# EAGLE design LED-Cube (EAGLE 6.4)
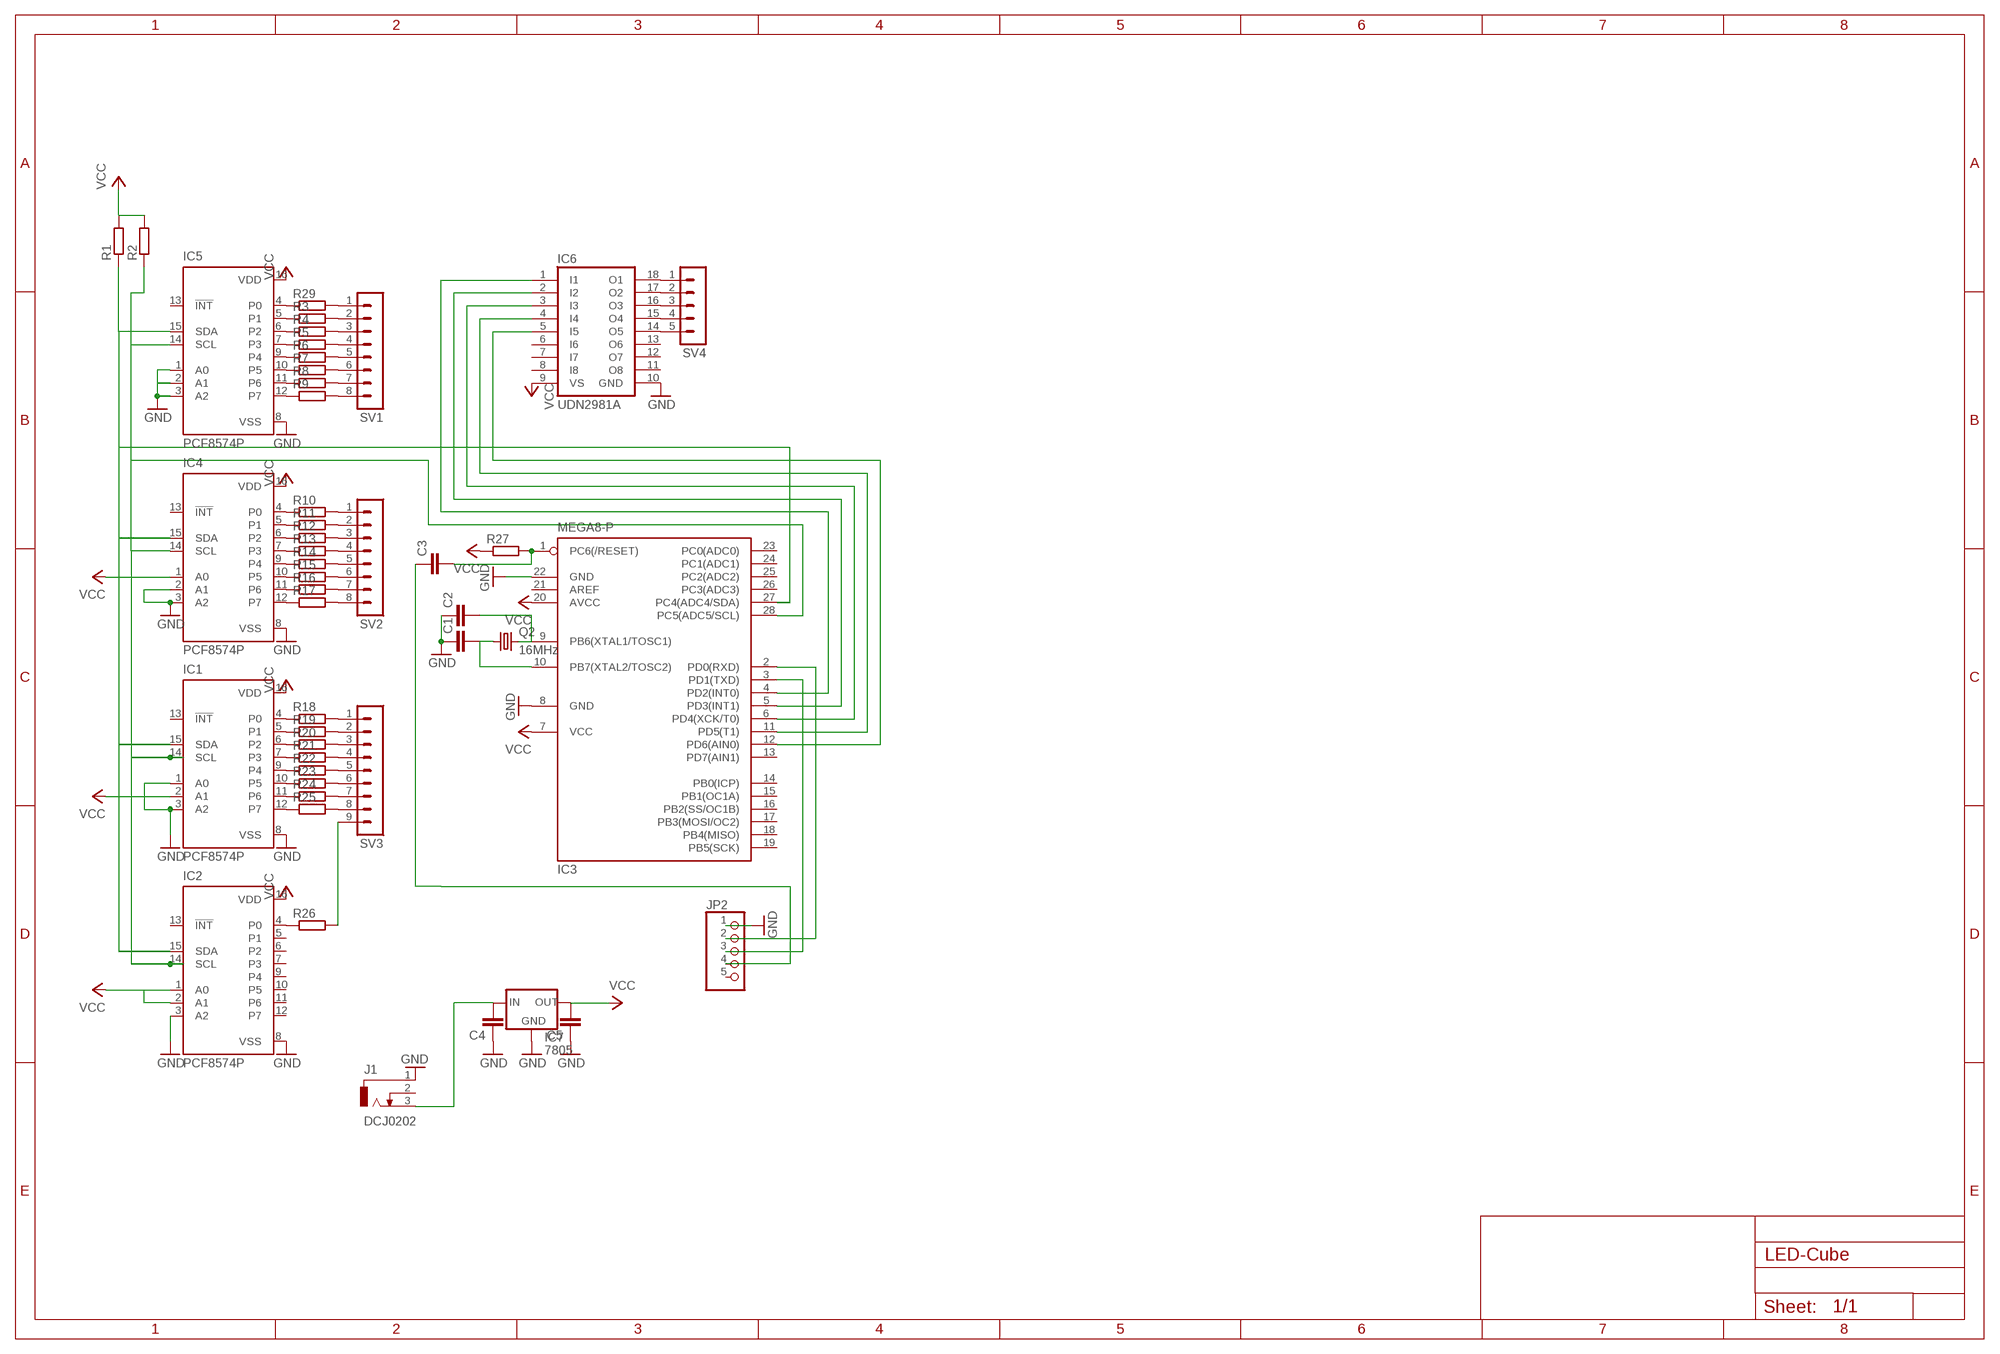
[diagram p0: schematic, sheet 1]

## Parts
C1  C-EU025-030X050  [C025-030X050]
C2  C-EU025-030X050  [C025-030X050]
C3  C-EU025-030X050  [C025-030X050]
C4  C-EU025-030X050  [C025-030X050]
C5  C-EU025-030X050  [C025-030X050]
IC1  PCF8574P  [DIL16]
IC2  PCF8574P  [DIL16]
IC3  MEGA8-P  [DIL28-3]
IC4  PCF8574P  [DIL16]
IC5  PCF8574P  [DIL16]
IC6  UDN2981A  [DIL18]
IC7  7805  V_REG_78XXSIDE  [78XXL]
J1  DCJ0202  [DCJ0202]
JP2  PINHD-1X5  [1X05]
Q2  16MHz  CRYSTALHC49S  [HC49/S]
R1  R-EU_0204/7  [0204/7]
R2  R-EU_0204/7  [0204/7]
R3  R-EU_0207/7  [0207/7]
R4  R-EU_0207/7  [0207/7]
R5  R-EU_0207/7  [0207/7]
R6  R-EU_0207/7  [0207/7]
R7  R-EU_0207/7  [0207/7]
R8  R-EU_0207/7  [0207/7]
R9  R-EU_0207/7  [0207/7]
R10  R-EU_0207/7  [0207/7]
R11  R-EU_0207/7  [0207/7]
R12  R-EU_0207/7  [0207/7]
R13  R-EU_0207/7  [0207/7]
R14  R-EU_0207/7  [0207/7]
R15  R-EU_0207/7  [0207/7]
R16  R-EU_0207/7  [0207/7]
R17  R-EU_0207/7  [0207/7]
R18  R-EU_0207/7  [0207/7]
R19  R-EU_0207/7  [0207/7]
R20  R-EU_0207/7  [0207/7]
R21  R-EU_0207/7  [0207/7]
R22  R-EU_0207/7  [0207/7]
R23  R-EU_0207/7  [0207/7]
R24  R-EU_0207/7  [0207/7]
R25  R-EU_0207/7  [0207/7]
R26  R-EU_0207/7  [0207/7]
R27  R-EU_0207/7  [0207/7]
R29  R-EU_0207/7  [0207/7]
SV1  MA08-1  [MA08-1]
SV2  MA08-1  [MA08-1]
SV3  MA09-1  [MA09-1]
SV4  MA05-1  [MA05-1]

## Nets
GND [GND]: C1.1 C2.1 C4.1 C5.1 IC1.1(A0) IC1.3(A2) IC1.8(VSS) IC2.3(A2) IC2.8(VSS) IC3.8(GND) IC3.22(GND) IC4.2(A1) IC4.3(A2) IC4.8(VSS) IC5.1(A0) IC5.2(A1) IC5.3(A2) IC5.8(VSS) IC6.10(GND) IC7.GND J1.1 JP2.1
N$1: IC1.14(SCL) IC2.14(SCL) IC3.28(PC5(ADC5/SCL)) IC4.14(SCL) IC5.14(SCL) R2.1
N$2: C3.1 JP2.4
N$3: IC5.4(P0) R29.1
N$4: R29.2 SV1.1
N$5: IC5.5(P1) R3.1
N$6: R3.2 SV1.2
N$7: IC5.6(P2) R4.1
N$8: R4.2 SV1.3
N$9: IC5.7(P3) R5.1
N$10: R5.2 SV1.4
N$11: IC5.10(P5) R7.1
N$12: R7.2 SV1.6
N$13: IC5.9(P4) R6.1
N$14: R6.2 SV1.5
N$15: IC5.11(P6) R8.1
N$16: R8.2 SV1.7
N$17: IC5.12(P7) R9.1
N$18: R9.2 SV1.8
N$19: IC4.4(P0) R10.1
N$20: R10.2 SV2.1
N$21: IC4.5(P1) R11.1
N$22: R11.2 SV2.2
N$23: IC4.6(P2) R12.1
N$24: R12.2 SV2.3
N$25: IC4.7(P3) R13.1
N$26: R13.2 SV2.4
N$27: IC4.9(P4) R14.1
N$28: R14.2 SV2.5
N$29: IC4.10(P5) R15.1
N$30: R15.2 SV2.6
N$31: IC4.11(P6) R16.1
N$32: R16.2 SV2.7
N$33: IC4.12(P7) R17.1
N$34: R17.2 SV2.8
N$35: IC1.4(P0) R18.1
N$36: R18.2 SV3.1
N$37: IC1.5(P1) R19.1
N$38: R19.2 SV3.2
N$39: IC1.6(P2) R20.1
N$40: R20.2 SV3.3
N$41: IC1.7(P3) R21.1
N$42: R21.2 SV3.4
N$43: IC1.9(P4) R22.1
N$44: R22.2 SV3.5
N$45: IC1.10(P5) R23.1
N$46: R23.2 SV3.6
N$47: IC1.11(P6) R24.1
N$48: R24.2 SV3.7
N$49: IC1.12(P7) R25.1
N$50: R25.2 SV3.8
N$51: IC2.4(P0) R26.1
N$52: R26.2 SV3.9
N$53: IC6.18(O1) SV4.1
N$54: IC6.17(O2) SV4.2
N$55: IC6.16(O3) SV4.3
N$56: IC6.15(O4) SV4.4
N$57: IC6.14(O5) SV4.5
N$59: IC3.3(PD1(TXD)) JP2.3
N$67: IC3.4(PD2(INT0)) IC6.1(I1)
N$68: IC3.5(PD3(INT1)) IC6.2(I2)
N$70: IC3.6(PD4(XCK/T0)) IC6.3(I3)
N$71: IC3.11(PD5(T1)) IC6.4(I4)
N$72: IC3.12(PD6(AIN0)) IC6.5(I5)
N$81: C3.2 IC3.1(PC6(/RESET)) R27.2
N$82: C2.2 IC3.9(PB6(XTAL1/TOSC1)) Q2.2
N$83: C1.2 IC3.10(PB7(XTAL2/TOSC2)) Q2.1
N$84: IC3.2(PD0(RXD)) JP2.2
N$86: C4.2 IC7.IN J1.3
N$88: IC1.15(SDA) IC2.15(SDA) IC3.27(PC4(ADC4/SDA)) IC4.15(SDA) IC5.15(SDA) R1.1
VCC [VCC]: C5.2 IC1.2(A1) IC1.16(VDD) IC2.1(A0) IC2.2(A1) IC2.16(VDD) IC3.7(VCC) IC3.20(AVCC) IC4.1(A0) IC4.16(VDD) IC5.16(VDD) IC6.9(VS) IC7.OUT R1.2 R2.2 R27.1
Unconnected: IC1.13(!INT) IC2.5(P1) IC2.6(P2) IC2.7(P3) IC2.9(P4) IC2.10(P5) IC2.11(P6) IC2.12(P7) IC2.13(!INT) IC3.13(PD7(AIN1)) IC3.14(PB0(ICP)) IC3.15(PB1(OC1A)) IC3.16(PB2(SS/OC1B)) IC3.17(PB3(MOSI/OC2)) IC3.18(PB4(MISO)) IC3.19(PB5(SCK)) IC3.21(AREF) IC3.23(PC0(ADC0)) IC3.24(PC1(ADC1)) IC3.25(PC2(ADC2)) IC3.26(PC3(ADC3)) IC4.13(!INT) IC5.13(!INT) IC6.6(I6) IC6.7(I7) IC6.8(I8) IC6.11(O8) IC6.12(O7) IC6.13(O6) J1.2 JP2.5

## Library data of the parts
C1-C5 = resistor:C-EU: CAPACITOR, European symbol
IC1 IC2 IC4 IC5 = micro-philips:PCF8574: I2C-Bus Remote 8-bit I/O expander http://www.semiconductors.philips.com/acrobat_download/datasheets/PCF8574_4.pdf; MPN: PCF8574PN; OC_FARNELL: 204020; OC_NEWARK: 11N8515
IC3 = atmel:MEGA8-P: MICROCONTROLLER 8 Kbytes FLASH, 1 kbytes SRAM, 512 bytes EEPROM, USART, 4-channel 10 bit ADC, 2-channel 8 bit ADC Pin compatible with Atmega48, ATMega88, ATMega168 Source: avr.lbr; OC_FARNELL: unknown; OC_NEWARK: unknown
IC6 = uln-udn:UDN298*: DRIVER ARRAY Source: Allegro Microsystems Inc. / UDN2981-UDN2984.pdf
IC7 = SparkFun:V_REG_78XX: Voltage Regulator Standard 7805 5V regulator. IGO (Input Ground Output). Spark Fun Electronics SKU : COM-00107
J1 = con-jack:DCJ0202: DC POWER JACK Source: DCJ0202.pdf; OC_FARNELL: unknown; OC_NEWARK: unknown
JP2 = pinhead:PINHD-1X5: PIN HEADER
Q2 = crystal:CRYSTAL: CRYSTAL; OC_FARNELL: 1667008; OC_NEWARK: unknown
R1 R2 = rcl:R-EU_: RESISTOR, European symbol
R3-R27 R29 = resistor:R-EU_: RESISTOR, European symbol
SV1 SV2 = con-lstb:MA08-1: PIN HEADER; OC_FARNELL: unknown; OC_NEWARK: unknown
SV3 = con-lstb:MA09-1: PIN HEADER; OC_FARNELL: unknown; OC_NEWARK: unknown
SV4 = con-lstb:MA05-1: PIN HEADER; OC_FARNELL: unknown; OC_NEWARK: unknown

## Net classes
1 VCC: width 0.508 mm
2 GND: width 0.508 mm

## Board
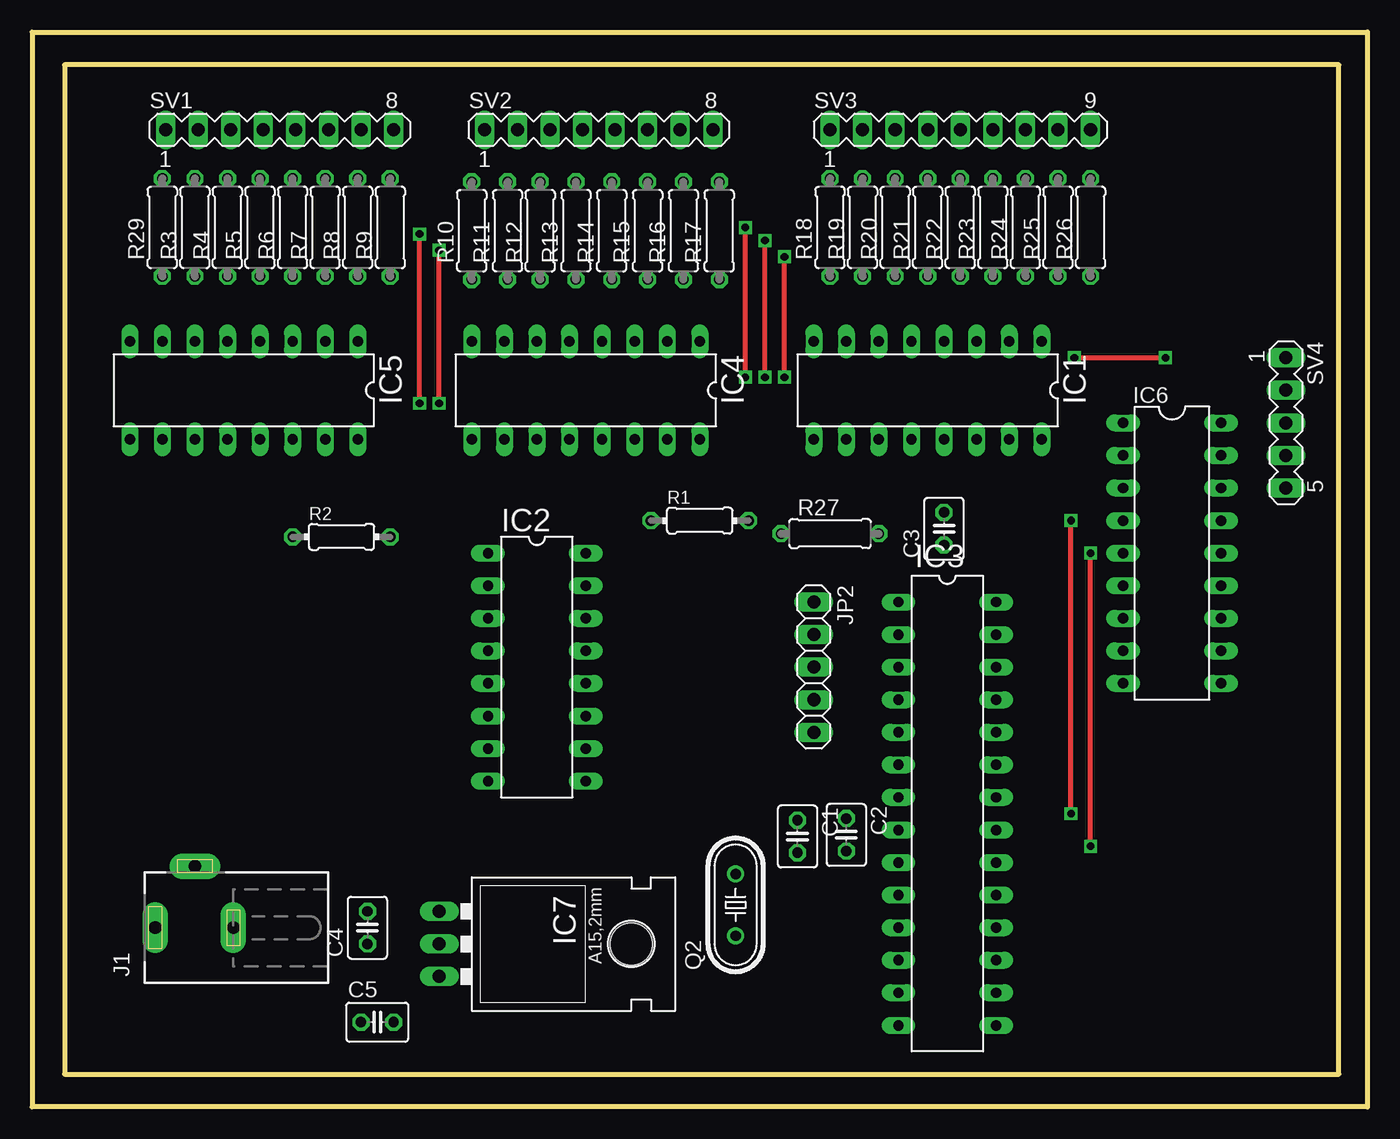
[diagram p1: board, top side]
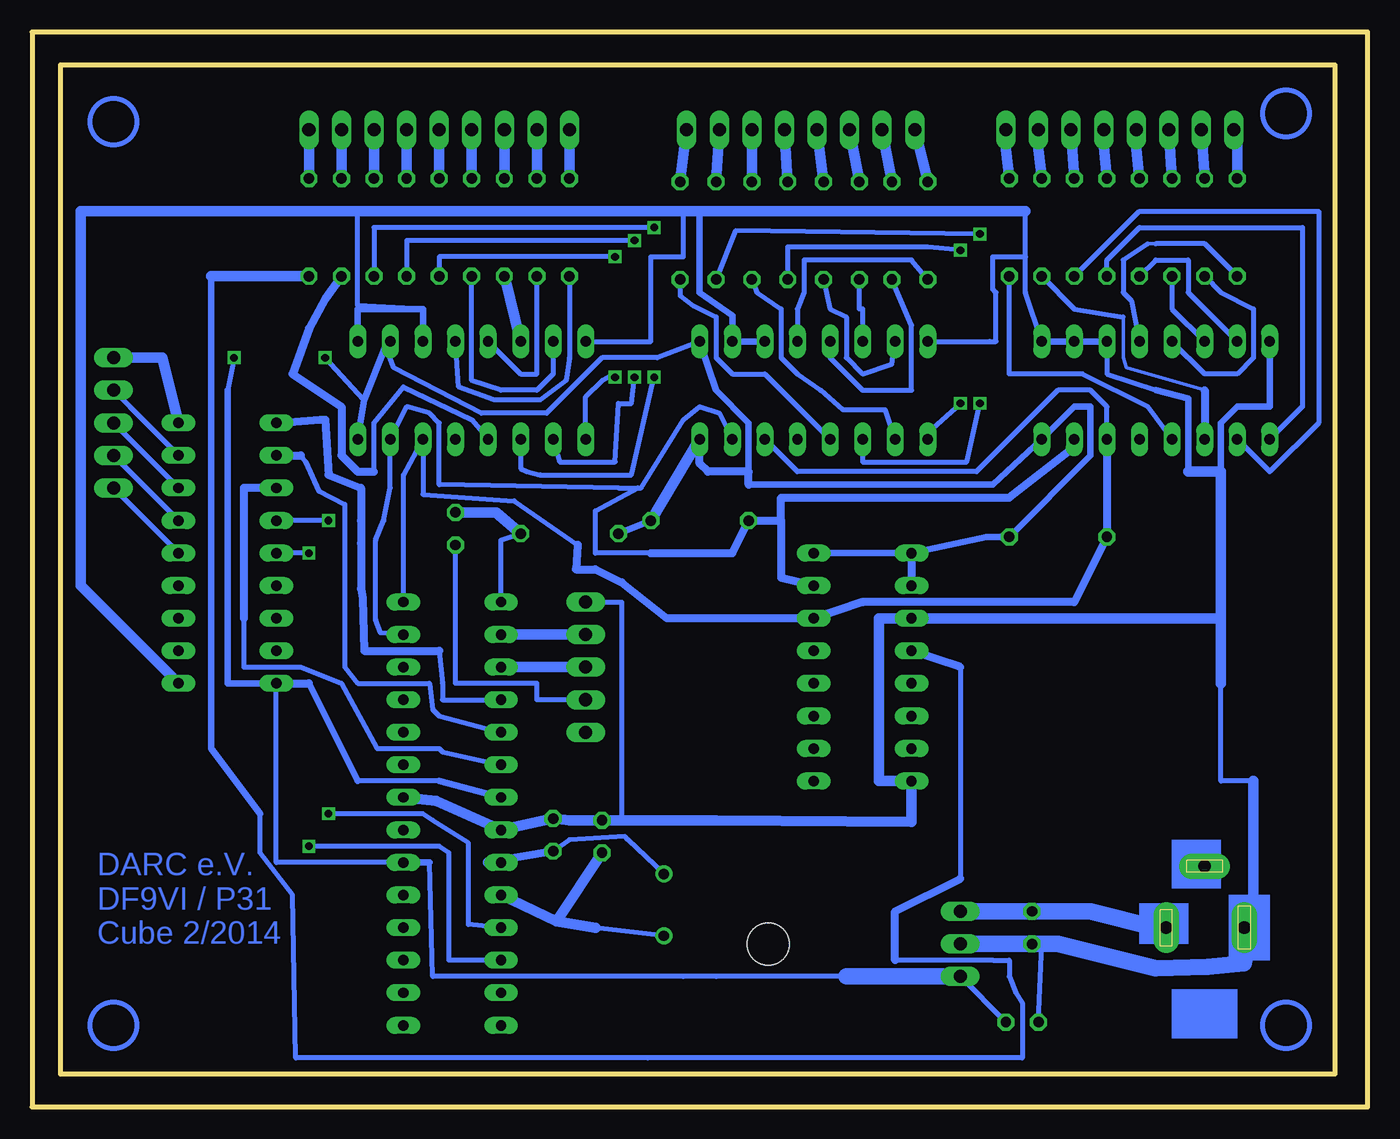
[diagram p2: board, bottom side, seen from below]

Size 104.14 x 83.82 mm. Coordinates in mm from the lower left corner, seen from the top.
Outline: 2.54,2.54 101.91,2.54 101.91,81.27 2.54,81.27 2.54,2.54
Outline: 0,83.82 104.14,83.82 104.14,0 0,0 0,83.82
Copper layers (1*16): Top 0.035mm / dielectric 1.5mm / Bottom 0.035mm
Design rules "default *": minimum track width 20mil, minimum drill 24mil, track to track 8mil, track to pad 8mil, pad to pad 8mil, via to via 8mil, smd to smd 8mil, copper to edge 40mil, drill to drill 8mil, minimum pad ring 10mil, minimum via ring 8mil, stop-mask expansion 4mil, vias tented up to drill 0mil, thermal gap 10mil
tRestrict: area 2.5,2.5 to 111.8,86.4

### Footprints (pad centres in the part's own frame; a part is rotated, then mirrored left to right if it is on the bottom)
C025-030X050 = drill 0.813 octagon: 1 -1.27,0; 2 1.27,0
DIL16 = drill 0.813 long: 1 -8.89,-3.81; 2 -6.35,-3.81; 3 -3.81,-3.81; 4 -1.27,-3.81; 5 1.27,-3.81; 6 3.81,-3.81; 7 6.35,-3.81; 8 8.89,-3.81; 9 8.89,3.81; 10 6.35,3.81; 11 3.81,3.81; 12 1.27,3.81; 13 -1.27,3.81; 14 -3.81,3.81; 15 -6.35,3.81; 16 -8.89,3.81
DIL28-3 = drill 0.813 long: 1 -16.51,-3.81; 2 -13.97,-3.81; 3 -11.43,-3.81; 4 -8.89,-3.81; 5 -6.35,-3.81; 6 -3.81,-3.81; 7 -1.27,-3.81; 8 1.27,-3.81; 9 3.81,-3.81; 10 6.35,-3.81; 11 8.89,-3.81; 12 11.43,-3.81; 13 13.97,-3.81; 14 16.51,-3.81; 15 16.51,3.81; 16 13.97,3.81; 17 11.43,3.81; 18 8.89,3.81; 19 6.35,3.81; 20 3.81,3.81; 21 1.27,3.81; 22 -1.27,3.81; 23 -3.81,3.81; 24 -6.35,3.81; 25 -8.89,3.81; 26 -11.43,3.81; 27 -13.97,3.81; 28 -16.51,3.81
DIL18 = drill 0.813 long: 1 -10.16,-3.81; 2 -7.62,-3.81; 3 -5.08,-3.81; 4 -2.54,-3.81; 5 0,-3.81; 6 2.54,-3.81; 7 5.08,-3.81; 8 7.62,-3.81; 9 10.16,-3.81; 10 10.16,3.81; 11 7.62,3.81; 12 5.08,3.81; 13 2.54,3.81; 14 0,3.81; 15 -2.54,3.81; 16 -5.08,3.81; 17 -7.62,3.81; 18 -10.16,3.81
78XXL = drill 1.016 long: GND 0,-3.81; IN -2.54,-3.81; OUT 2.54,-3.81 | hole 3.302: 0,11.176
DCJ0202 = drill 1 pad 2 long: 1 0,3.1; 2 4.8,0; 3 0,-3
1X05 = drill 1.016 long: 1 -5.08,0; 2 -2.54,0; 3 0,0; 4 2.54,0; 5 5.08,0
HC49/S = drill 0.813: 1 -2.413,0; 2 2.413,0
0204/7 = drill 0.813 octagon: 1 -3.81,0; 2 3.81,0
0207/7 = drill 0.813 octagon: 1 -3.81,0; 2 3.81,0
MA08-1 = drill 1.016 long: 1 -8.89,0; 2 -6.35,0; 3 -3.81,0; 4 -1.27,0; 5 1.27,0; 6 3.81,0; 7 6.35,0; 8 8.89,0
MA09-1 = drill 1.016 long: 1 -10.16,0; 2 -7.62,0; 3 -5.08,0; 4 -2.54,0; 5 0,0; 6 2.54,0; 7 5.08,0; 8 7.62,0; 9 10.16,0
MA05-1 = drill 1.016 long: 1 -5.08,0; 2 -2.54,0; 3 0,0; 4 2.54,0; 5 5.08,0

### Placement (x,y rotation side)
C1  59.69,21.08 270 top
C2  63.5,21.21 270 top
C3  71.12,45.09 90 top
C4  26.16,13.97 90 top
C5  26.92,6.6 0 top
IC1  69.85,55.88 180 top
IC2  39.37,34.29 270 top
IC3  71.37,22.86 270 top
IC4  43.18,55.88 180 top
IC5  16.51,55.88 180 top
IC6  88.9,43.18 270 top
IC7  35.56,12.7 270 top
J1  12.7,13.97 90 top
JP2  60.96,34.29 270 top
Q2  54.86,15.75 90 top
R1  52.07,45.72 0 top
R2  24.13,44.45 0 top
R3  12.7,68.58 90 top
R4  15.24,68.58 90 top
R5  17.78,68.58 90 top
R6  20.32,68.58 90 top
R7  22.86,68.58 90 top
R8  25.4,68.58 90 top
R9  27.94,68.58 90 top
R10  34.29,68.33 90 top
R11  37.08,68.33 90 top
R12  39.62,68.33 90 top
R13  42.42,68.33 90 top
R14  45.21,68.33 90 top
R15  48.01,68.33 90 top
R16  50.8,68.33 90 top
R17  53.59,68.33 90 top
R18  62.23,68.58 90 top
R19  64.77,68.58 90 top
R20  67.31,68.58 90 top
R21  69.85,68.58 90 top
R22  72.39,68.58 90 top
R23  74.93,68.58 90 top
R24  77.47,68.58 90 top
R25  80.01,68.58 90 top
R26  82.55,68.58 90 top
R27  62.23,44.7 0 top
R29  10.16,68.58 90 top
SV1  19.3,76.2 0 top
SV2  44.2,76.2 0 top
SV3  72.39,76.2 0 top
SV4  97.79,53.34 270 top

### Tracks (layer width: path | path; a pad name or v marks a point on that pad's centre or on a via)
GND
  Bottom 0.406: IC5.3 20.32,57.15 16.51,55.88 | IC5.1 26.67,63.5 26.67,66.29 | 26.67,66.29 26.67,69.85 | C4.1 25.4,12.7 C5.1 | 8.89,25.4 11.43,25.4 11.43,33.02 | C1.1 C2.1 | JP2.1 58.17,39.37 58.17,22.35 | IC4.8 29.46,59.69 28.96,59.69 28.96,63.5 29.21,63.75 29.21,66.29 26.67,66.29 | IC1.8 55.88,59.69 55.88,66.29 53.34,66.29 53.34,69.85 | 73.66,62.23 78.74,62.48 78.74,69.85
  Bottom 0.508: IC4.3 IC4.2 49.53,61.72 52.07,63.5 52.07,69.85 | IC5.3 IC5.2 IC5.1 | IC1.3 73.66,62.23 78.74,62.23 IC1.1 | IC5.8 7.62,54.61 10.16,54.61 11.43,53.34 11.43,49.53 | 16.51,55.88 13.97,55.24 13.97,49.53 | 8.89,13.97 J1.1 8.89,13.97
  Bottom 0.813: IC6.10 100.33,40.64 100.33,69.85 78.74,69.85 73.66,69.85 58.42,69.85 55.88,69.85 53.34,69.85 52.07,69.85 34.29,69.85 28.96,69.85 26.67,69.85 | IC3.22 72.64,23.88 IC3.8 C2.1 62.23,22.35 58.17,22.35 54.1,22.35 51.31,22.35 50.8,22.35 35.56,22.22 IC2.8 38.1,25.4 38.1,30.48 38.1,38.1 IC2.3 11.43,38.1 | 11.43,33.02 11.43,38.1 | 11.43,38.1 11.43,49.53 13.97,49.53 | 8.89,25.4 8.89,13.97
  Bottom 1.27: 8.89,13.97 9.65,11.18 12.45,10.92 16.51,10.8 24.13,12.7 25.4,12.7 C4.1 IC7.GND
N$1
  Bottom 0.406: IC4.14 44.45,49.53 30.48,49.53 24.13,55.88 21.59,55.88 20.32,54.61 IC5.14 | IC3.28 75.18,49.28 IC1.14 73.66,47.75 66.55,47.24 61.59,43.81
  Bottom 0.61: IC5.14 R2.1 22.86,39.37 39.37,39.37 IC2.14 54.61,38.1 58.17,40.89 60.2,41.91 61.72,41.91 61.59,43.81
N$2
  Bottom 0.406: JP2.4 64.77,31.75 64.77,32.77 64.77,33.02 71.12,33.02 C3.1
N$3
  Bottom 0.254: 16.51,67.31 17.14,67.31
  Bottom 0.406: IC5.4 18.41,62.87 19.05,63.5 19.05,66.04 17.14,67.31 | 16.51,67.31 12.7,67.31 R29.1
N$4
  Bottom 0.406: SV1.1 10.16,76.2
  Bottom 0.813: 10.16,76.2 R29.2
N$5
  Bottom 0.406: IC5.5 12.7,57.15 10.16,57.15 8.89,58.42 8.89,62.23 11.43,63.5 R3.1
N$6
  Bottom 0.813: SV1.2 R3.2
N$7
  Bottom 0.406: IC5.6 15.24,62.23 R4.1
N$8
  Bottom 0.813: SV1.3 R4.2
N$9
  Bottom 0.406: IC5.7 13.97,63.5 13.97,66.04 16.51,66.04 R5.1
N$10
  Bottom 0.813: R5.2 18.03,74.68 SV1.4
N$11
  Bottom 0.406: IC5.10 7.62,49.53 3.81,53.34 3.81,69.85 17.78,69.85 R7.1
N$12
  Bottom 0.813: SV1.6 R7.2
N$13
  Bottom 0.406: IC5.9 5.08,54.61 5.08,68.58 17.78,68.58 20.32,66.04 R6.1
N$14
  Bottom 0.813: R6.2 20.57,74.93 SV1.5
N$15
  Bottom 0.254: 12.7,55.88 18.8,57.66 19.05,58.42 19.05,61.59
  Bottom 0.406: 19.05,61.59 22.86,62.23 R8.1
  Bottom 0.61: 12.7,55.88 IC5.11
N$16
  Bottom 0.813: R8.2 25.65,74.68 SV1.7
N$17
  Bottom 0.406: IC5.12 17.14,54.61 22.22,57.15 27.94,57.15 R9.1
N$18
  Bottom 0.813: R9.2 28.19,74.68 SV1.8
N$19
  Bottom 0.406: IC4.4 44.45,62.23 43.94,63.5 43.94,66.04 38.1,66.04 35.56,66.04 R10.1
N$20
  Bottom 0.813: R10.2 SV2.1
N$21
  Bottom 0.254: IC4.5 41.91,58.42
  Bottom 0.406: R11.1 35.56,60.96 35.56,55.88 39.37,55.88 41.91,58.42
N$22
  Bottom 0.813: R11.2 SV2.2
N$23
  Bottom 0.406: IC4.6 39.37,62.23 39.62,62.23 R12.1
N$24
  Bottom 0.813: R12.2 SV2.3
N$25
  Bottom 0.406: IC4.7 37.08,57.91 39.37,57.15 40.64,58.42 40.64,61.59 41.91,62.23 R13.1
N$26
  Bottom 0.813: R13.2 SV2.4
N$27  (via drill 0.6)
  Top 0.406: v31.75,54.86 v31.75,66.8
  Bottom 0.406: IC4.9 34.29,52.58 v31.75,54.86 | v31.75,66.8 34.29,67.06 45.21,67.06 R14.1
N$28
  Bottom 0.813: R14.2 SV2.5
N$29
  Bottom 0.406: R15.1 47.62,63.5 45.72,62.23 45.72,58.42 44.45,57.15 42.67,55.88 40.89,54.36 37.59,54.36 IC4.10
N$30
  Bottom 0.813: R15.2 SV2.6
N$31  (via drill 0.6)
  Top 0.406: v30.23,54.86 v30.23,68.07
  Bottom 0.406: IC4.11 39.37,50.29 31.24,50.29 v30.23,54.86 | v30.23,68.07 49.28,68.33 R16.1
N$32
  Bottom 0.813: R16.2 SV2.7
N$33
  Bottom 0.406: IC4.12 46.99,57.15 49.53,57.15 50.8,58.42 50.8,61.59 52.58,62.48 53.59,63.25 R17.1
N$34
  Bottom 0.813: R17.2 SV2.8
N$35
  Bottom 0.406: IC1.4 70.87,56.13 68.07,55.12 64.52,55.12 62.48,56.64 62.23,58.42 R18.1
N$36
  Bottom 0.813: R18.2 SV3.1
N$37
  Bottom 0.406: R19.1 64.77,57.15 66.04,57.15 IC1.5
N$38
  Bottom 0.813: R19.2 SV3.2
N$39
  Bottom 0.813: IC1.6 R20.1
N$40
  Bottom 0.813: R20.2 SV3.3
N$41
  Bottom 0.406: IC1.7 63.5,57.15 64.77,55.88 67.56,55.88 69.85,56.64 R21.1
N$42
  Bottom 0.813: R21.2 SV3.4
N$43  (via drill 0.6)
  Top 0.406: v58.67,56.9 v58.67,66.29
  Bottom 0.406: IC1.9 60.96,55.37 59.69,56.64 59.18,56.9 v58.67,56.9 | v58.67,66.29 72.39,66.29 R22.1
N$44
  Bottom 0.813: R22.2 SV3.5
N$45  (via drill 0.6)
  Top 0.406: v57.15,56.9 v57.15,67.56
  Bottom 0.406: IC1.10 62.99,50.29 58.67,50.29 58.42,54.86 57.4,54.86 v57.15,56.9 | v57.15,67.56 74.93,67.56 R23.1
N$46
  Bottom 0.813: R23.2 SV3.6
N$47  (via drill 0.6)
  Top 0.406: v55.63,56.9 v55.63,68.58
  Bottom 0.406: IC1.11 66.04,49.78 65.53,49.53 64.52,49.28 57.4,49.28 v55.63,56.9 | v55.63,68.58 77.47,68.58 R24.1
N$48
  Bottom 0.813: R24.2 SV3.7
N$49
  Bottom 0.406: IC1.12 69.85,53.59 75.18,56.13 77.47,53.34 77.47,49.53
  Bottom 0.61: 77.47,49.53 78.74,49.53 80.01,50.8 80.01,54.61 83.82,57.15 82.55,60.71 81.28,62.99 R25.1
N$50
  Bottom 0.813: R25.2 SV3.8
N$51
  Bottom 0.406: 36.83,11.43 29.21,11.43 27.94,11.43 27.94,10.16 27.43,8.89 26.92,8.13 26.92,3.81 56.13,3.81 83.57,3.81 83.82,16.51 86.36,19.81 86.36,22.86 | 31.75,34.29 31.75,17.78
  Bottom 0.508: 86.36,22.86 90.17,27.94 90.17,64.77
  Bottom 0.61: 31.75,34.29 IC2.4 | 31.75,17.78 36.83,15.24 36.83,11.43
  Bottom 0.813: R26.1 90.17,64.77
N$52
  Bottom 0.813: R26.2 SV3.9
N$53
  Bottom 0.813: IC6.18 93.98,58.42 SV4.1
N$54
  Bottom 0.406: SV4.2 96.52,54.61 IC6.17
N$55
  Bottom 0.406: SV4.3 IC6.16
N$56
  Bottom 0.406: SV4.4 IC6.15
N$57
  Bottom 0.406: SV4.5 IC6.14
N$59
  Bottom 0.813: JP2.3 IC3.3
N$67
  Bottom 0.406: IC3.4 72.14,31.75 72.14,33.02 72.39,35.56
  Bottom 0.61: 72.39,35.56 78.23,35.56 78.36,39.62 78.49,40.39 78.49,43.94 78.49,45.72 78.49,48.26 81.03,49.28 81.28,53.59 81.66,53.59 IC6.1
N$68
  Bottom 0.406: IC3.5 72.39,30.48 72.9,30.99 73.15,33.02 78.74,33.02 79.76,34.29 79.76,46.99 81.79,48.01 82.8,50.29 83.19,50.8
  Bottom 0.61: IC6.2 83.19,50.8
N$70
  Bottom 0.406: IC3.6 72.14,27.69 72.39,27.94 77.22,27.94 80.01,33.02 83.19,34.29 87.63,34.29 87.63,38.1
  Bottom 0.61: 87.63,38.1 87.63,48.26 IC6.3
N$71  (via drill 0.6)
  Top 0.406: v81.03,22.86 v81.03,45.72
  Bottom 0.406: IC3.11 70.1,14.22 70.1,20.57 72.9,22.35 73.66,22.86 v81.03,22.86 | v81.03,45.72 IC6.4
N$72  (via drill 0.6)
  Top 0.406: v82.55,20.32 v82.55,43.18
  Bottom 0.406: IC3.12 71.63,11.43 71.63,19.81 72.39,20.32 v82.55,20.32 | v82.55,43.18 IC6.5
N$81
  Bottom 0.406: IC3.1 67.56,44.2 R27.2
  Bottom 0.813: C3.2 67.95,46.35 R27.2
N$82
  Bottom 0.406: 68.58,19.05 C2.2 62.23,20.83 57.91,21.08 57.66,20.83 Q2.2
  Bottom 0.61: C2.2 68.58,19.05
  Bottom 0.813: IC3.9 68.58,19.05
N$83
  Bottom 0.406: Q2.1 60.2,13.97
  Bottom 0.813: 63.25,14.48 60.2,13.97 | IC3.10 63.25,14.48 | 63.25,14.48 C1.2
N$84
  Bottom 0.813: JP2.2 IC3.2
N$86
  Bottom 0.254: 15.24,13.97 J1.3 16.51,13.97
  Bottom 0.406: C4.2 27.94,15.24
  Bottom 1.27: 16.51,13.97 21.59,15.24 C4.2 IC7.IN
N$88
  Bottom 0.406: IC4.15 50.55,54.1 52.07,54.61 53.34,53.59 56.64,48.26 56.9,48.26 | 56.9,48.26 58.42,48.26 72.39,48.51 72.39,53.34 73.15,54.1 74.93,54.61 IC1.15 76.2,48.26 76.71,45.72 77.34,44.2 77.34,37.97 76.96,36.96 IC3.27 | 55.88,43.18 60.2,43.18 60.2,46.48 56.9,48.26
  Bottom 0.61: 45.72,45.72 45.72,41.27 IC2.15 | 45.72,45.72 R1.1 49.53,43.18 55.88,43.18 | IC5.15 22.86,51.44 27.94,47.5 45.72,47.5 45.72,45.72
VCC  (via drill 0.6)
  Top 0.406: v81.28,58.42 v88.39,58.42
  Bottom 0.406: C5.2 IC7.OUT | 50.8,10.16 53.34,10.16 | 53.34,10.16 72.9,10.16 73.15,19.05 85.09,19.05 IC6.9 | 40.64,10.16 53.34,10.16 | 72.39,25.4 78.74,25.4 | IC4.1 55.37,58.42 59.69,58.42 64.01,54.1 69.09,54.1 75.95,57.66 76.58,59.31 | 78.23,55.12 v81.28,58.42 | v88.39,58.42 88.9,55.88
  Bottom 0.508: IC2.16 IC2.1 29.72,44.45 R2.2 21.59,50.8 21.59,54.61 22.86,54.61 IC5.16 29.21,48.51 48.26,48.51 | IC1.16 78.23,55.12 76.58,59.31 IC1.2 | R27.1 R1.2 | IC4.1 50.8,55.88 48.26,53.34 48.26,49.53 | 82.55,33.02 78.74,25.4 | 72.39,25.4 IC3.7 | 73.15,19.05 IC3.20 | 88.9,55.88 88.9,33.02 IC6.9
  Bottom 0.61: IC2.1 IC2.2 | IC6.9 82.55,33.02 | 48.26,48.51 48.26,49.53 51.44,49.53 52.07,50.16 IC4.16
  Bottom 0.813: R1.2 IC4.16
  Bottom 1.27: IC7.OUT 40.64,10.16
(copper drawn outside any net)
  shapes: Bottom area x4, Bottom circle x4

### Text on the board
Bottom: DARC e.V. / DF9VI / P31 / Cube 2/2014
